(* 
1、电机安全地址设置：5个电机，从1到5的安全地址分别是 100~104
2、FSOE connection 从200开始

 *)
PROGRAM MAIN
VAR
	AxisDrive_1		:	ARRAY[0..4] OF ST_ToAmp8000;
	Axis1			:	AXIS_REF;
	fbPower			:	MC_Power;
	fbMovAbs		:	MC_MoveAbsolute;
	bEnable			:	BOOL;
	bRun			:	BOOL;
END_VAR

//AxisDrive_1[0].STO_Activate := TRUE;

fbPower(
	Axis:= Axis1, 
	Enable:= bEnable, 
	Enable_Positive:= TRUE, 
	Enable_Negative:= TRUE, 
	Override:= 100, 
	BufferMode:= , 
	Options:= , 
	Status=> , 
	Busy=> , 
	Active=> , 
	Error=> , 
	ErrorID=> );
fbMovAbs(
	Axis:= Axis1, 
	Execute:= bRun, 
	Position:= 1000, 
	Velocity:= 200, 
	Acceleration:= , 
	Deceleration:= , 
	Jerk:= , 
	BufferMode:= , 
	Options:= , 
	Done=> , 
	Busy=> , 
	Active=> , 
	CommandAborted=> , 
	Error=> , 
	ErrorID=> );

END_PROGRAM
